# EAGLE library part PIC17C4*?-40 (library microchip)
MICROCONTROLLER EPROM-based
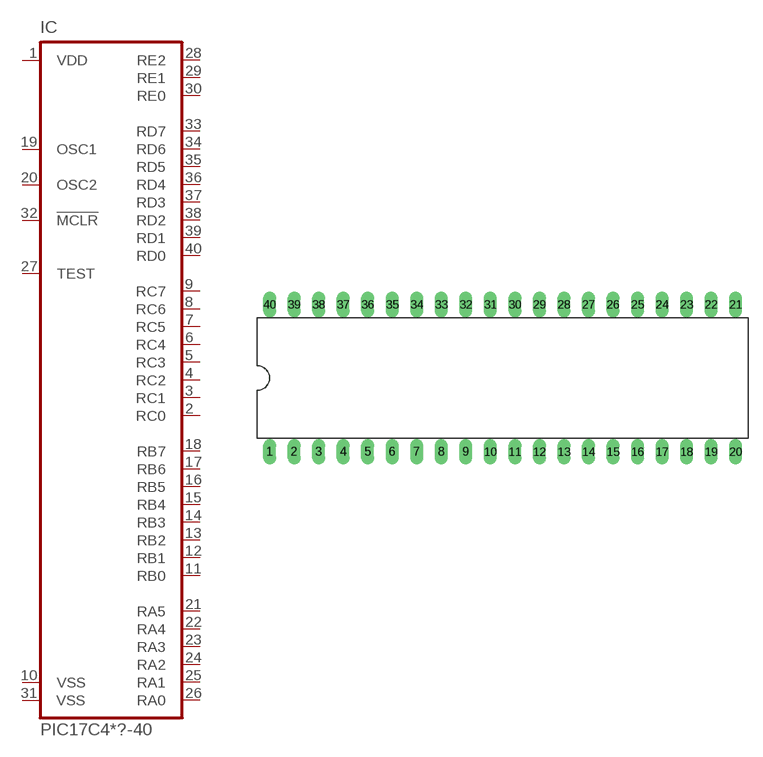
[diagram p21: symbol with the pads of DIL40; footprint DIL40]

Designator prefix IC

## PIC17C42P-40 (MF: MICROCHIP; MPN: PIC17C42A-16/P; OC_FARNELL: 1196768; OC_NEWARK: 23C5768), PIC17C43P-40 (MF: MICROCHIP; MPN: PIC17C43-16/P; OC_FARNELL: 1084356; OC_NEWARK: 63K6089), PIC17C44P-40 (MF: MICROCHIP; MPN: PIC17C44-33/P; OC_FARNELL: 1084221; OC_NEWARK: 23C5919)  [DIL40]
1  VDD  pwr
2  RC0  out
3  RC1  out
4  RC2  out
5  RC3  out
6  RC4  out
7  RC5  out
8  RC6  out
9  RC7  out
10  VSS  pwr
11  RB0
12  RB1
13  RB2
14  RB3
15  RB4
16  RB5
17  RB6
18  RB7
19  OSC1  in
20  OSC2  out
21  RA5
22  RA4
23  RA3
24  RA2
25  RA1
26  RA0
27  TEST  in
28  RE2
29  RE1
30  RE0
31  VSS  pwr
32  !MCLR  in
33  RD7
34  RD6
35  RD5
36  RD4
37  RD3
38  RD2
39  RD1
40  RD0

## Footprint DIL40 (pad centres in mm)
Dual In Line package type P
drill 0.813 long: 1 -24.13,-7.62; 2 -21.59,-7.62; 3 -19.05,-7.62; 4 -16.51,-7.62; 5 -13.97,-7.62; 6 -11.43,-7.62; 7 -8.89,-7.62; 8 -6.35,-7.62; 9 -3.81,-7.62; 10 -1.27,-7.62; 11 1.27,-7.62; 12 3.81,-7.62; 13 6.35,-7.62; 14 8.89,-7.62; 15 11.43,-7.62; 16 13.97,-7.62; 17 16.51,-7.62; 18 19.05,-7.62; 19 21.59,-7.62; 20 24.13,-7.62; 21 24.13,7.62; 22 21.59,7.62; 23 19.05,7.62; 24 16.51,7.62; 25 13.97,7.62; 26 11.43,7.62; 27 8.89,7.62; 28 6.35,7.62; 29 3.81,7.62; 30 1.27,7.62; 31 -1.27,7.62; 32 -3.81,7.62; 33 -6.35,7.62; 34 -8.89,7.62; 35 -11.43,7.62; 36 -13.97,7.62; 37 -16.51,7.62; 38 -19.05,7.62; 39 -21.59,7.62; 40 -24.13,7.62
